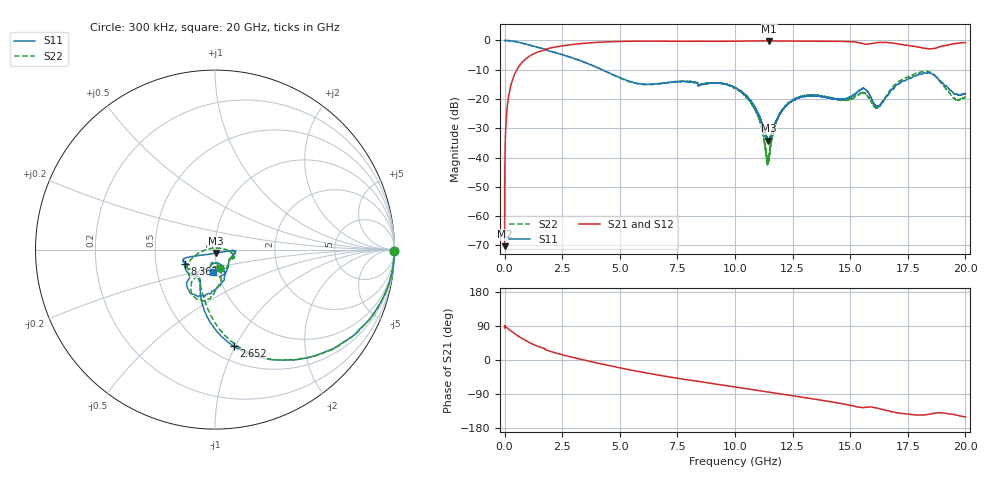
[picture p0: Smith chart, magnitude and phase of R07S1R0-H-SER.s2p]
!{R07S1R0}
!Johanson Technology Inc.
!www.johansontechnology.com
!Test Board Conditions:
!Substrate Type  RO4350B
!Substrate Thickness  10 mil
!Substrate Dk  3.66
!TL Type: GCPW
!TL Trace Width  21 mil
!TL Gap  20 mil
!Electrode orientation  Horizontal
!DUT TOPOLOGY	SERIES
!Mounting Pad LxW  16x21 mil
! Created Fri Feb  5 23:08:36 2021
# hz S ma R 50
! 2 Port Network Data from SP1.SP block
! freq  magS11  angS11  magS21  angS21  magS12  angS12  magS22  angS22
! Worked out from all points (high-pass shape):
!   20001 points, 300 kHz to 20 GHz, reference 50 ohm
!   highest |S21| = -0.14 dB at 11.48 GHz (marker M1); lowest = -70.3 dB at 300 kHz (marker M2)
!   |S21| within 3 dB of the highest: 1.75 GHz to end of sweep
!   lowest |S11| = -34.3 dB at 11.45 GHz (marker M3), VSWR 1.04, Z = 50.3 - j1.91 ohm
!   |S11| at or under -10 dB: 4.235 GHz to end of sweep
!   |S22| runs from -42.6 to 0.0 dB; largest |S21 - S12| = 0.01
!   S11 on the Smith chart (normalised r, x): 300 kHz: open; 2.652 GHz: 0.64, -0.99; 8.367 GHz: 0.71, -0.12; 20 GHz: 0.95, -0.24
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300000  0.9971 -0.3  0.0003054 84.5  0.0001458 103.1  1 -0.3
1.203e8  0.9957 -5.7  0.07737 84.2  0.07739 84.1  0.9964 -5.7
4.073e8  0.9657 -18.7  0.2491 70.7  0.248 70.6  0.9649 -18.9
1.2503e9  0.7991 -48.5  0.5887 41.1  0.5873 41.0  0.802 -48.4
2.6523e9  0.5481 -79.1  0.8255 11.4  0.824 11.5  0.5492 -77.3
3.3343e9  0.4436 -90.0  0.886 1.3  0.8852 1.4  0.4451 -86.8
6.6673e9  0.1822 -125.3  0.9717 -39.7  0.972 -39.7  0.1812 -132.0
8.3673e9  0.1854 -153.7  0.9664 -56.2  0.9677 -56.1  0.19 -136.2
1.00003e10  0.1581 -164.0  0.9712 -71.2  0.9732 -71.2  0.153 -156.2
1.08903e10  0.06904 -154.2  0.9817 -79.4  0.9796 -79.4  0.06322 -175.2
1.14463e10  0.01933 -79.8  0.9812 -84.6  0.9817 -84.6  0.008972 75.6
1.14833e10  0.02037 -68.4  0.9835 -84.9  0.9815 -84.9  0.01039 53.7
1.17393e10  0.03766 -22.0  0.9804 -87.4  0.9814 -87.3  0.03465 8.7
1.20883e10  0.06697 -7.0  0.9777 -90.5  0.9793 -90.6  0.0678 -2.6
1.33343e10  0.1146 -6.7  0.9712 -102.2  0.9702 -102.2  0.1169 -23.1
1.47323e10  0.09925 -37.2  0.9639 -116.5  0.9633 -116.5  0.09503 -31.5
1.55803e10  0.1519 -81.3  0.8756 -125.6  0.8759 -125.5  0.1269 -78.1
1.61403e10  0.07488 -91.1  0.9163 -126.5  0.9152 -126.5  0.07009 -94.7
1.66673e10  0.1202 -65.2  0.9097 -134.0  0.9126 -134.4  0.1306 -75.1
1.83273e10  0.2759 -114.2  0.7251 -144.2  0.7236 -144.3  0.2969 -108.5
1.95353e10  0.1206 -116.6  0.8812 -144.4  0.8836 -144.6  0.1006 -102.3
2e10  0.1236 -94.0  0.9221 -150.6  0.9202 -150.6  0.108 -74.8
